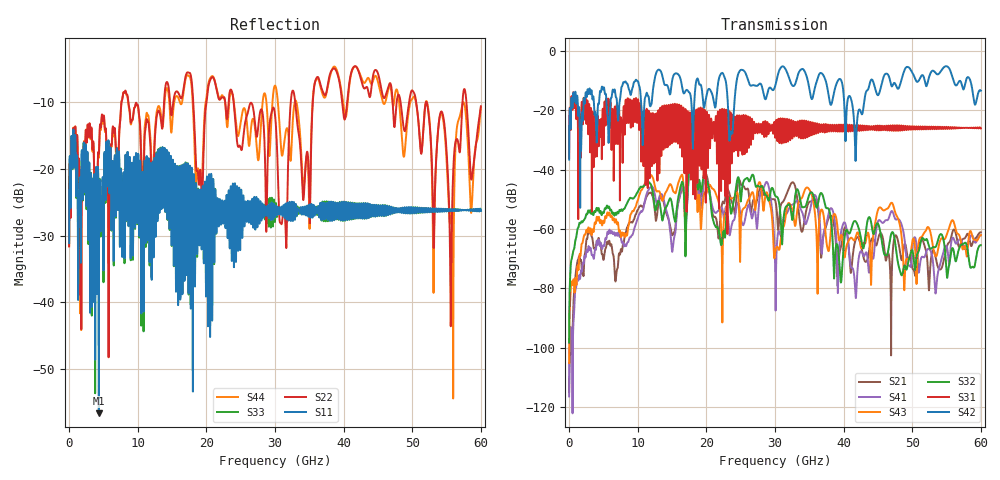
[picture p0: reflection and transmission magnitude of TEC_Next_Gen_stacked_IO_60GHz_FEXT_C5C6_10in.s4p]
!! CHANNEL DESCRIPTION:  Next Generation 28Gbps Press-fit Stacked I/O Connector
!!  with 10" 5-6-5 Megtron 6 Stripline trace on host side and 1.25" 7-5-7 Megtron 6 Microstrip trace on plug side
!! HOST PCB DESCRIPTION:  PCB thickness 3.425 mm
!!  26 Layer Board, 15 GND planes, 4 Layer route-out on Layers 7,11,17,21, 8mil stub on vias
!!  Pairs on following layers
!!  Layer 07 - A02A03 A14A15 D05D06
!!  Layer 11 - D020D3 C05C06 D14D15
!!  Layer 17 - C02C03 B05B06 C14C15
!!  Layer 21 - B02B03 A05A06 B14B15
!! CONNECTOR DESCRIPTION:  Next Generation 28Gbps Press-fit Stacked I/O Connector
!! PLUG-IN CARD DESCRIPTION:  PCB thickness 1mm thick
!!  6 Layer Board, 4 GND planes, 0.35 x 1.4mm mating pads
!!  Micro-strip diff traces referenced to GND plane 3mils down, 2nd GND plane 17mils from top of board
!!  PCB GND planes are symmetric
!! MODEL DESCRIPTION: TE Connectivity S-parameter model produced from Macro-model, Extracted .s4p FEXT (Victim B05B06 - Aggressor C05C06)
!! MODEL DATE: 5/15/2014 CR32f, FPR23
!! MODEL STATUS: Developmental
!! MODEL GEOMETRY: 4 Rows - Rows A, B, C, D. 3 pairs in each row, 12 total pairs
!! MODEL FREQUENCY RANGE: DC to 60 GHz in 10 MHz frequency steps
!! MODEL EDGE RATE LIMITATION: 8.33 ps (Using conservative 0.5/Fmax rule of thumb)
!! TIME-DOMAIN TRANSFORM CAUTIONS:
!! 1.) Do not simulate transient edge rates faster than the number listed above.  Edge
!!  rates faster than this number contain significant spectral content at frequencies
!!  above the model's highest frequency.
!! 2.) Even when simulating edge rates that are slower than the number listed above, be
!!  aware that the best time resolution possible with a direct iFFT is (1 / 2Fmax).
!!  As a result, time resolution is typically not adequate for most time-domain
!!  simulations unless tricks such as frequency-domain zero-padding and windowing are
!!  used to minimize leakage and aliasing.
!! 3.) Because the model has a uniform frequency step, a direct iFFT will result in an
!!  impulse that that has a time length given by either (1 / Fstep) or (1 / 2Fstep),
!!  depending on the transform being used.  Care has been taken in selecting the
!!  frequency step to ensure a settled impulse response for the model.  Therefore,
!!  convolution with the model's impulse response should present no issues.  However,
!!  if directly concatenating s-parameter models in the frequency domain a user must
!!  either interpolate necessary interim frequencies or complete impulse response
!!  zero-padding.  Impulse response zero-padding is more difficult, but more accurate.
!! PORT DEFINITIONS:
!! Port  1  ----->  Host C05		B05 Module <-----  Port  2
!! Port  3  ----->  Host C06		B06 Module <-----  Port  4
!! Touchstone data
! Created: 29-Sep-2014 by IdEM R2011 (7.0.3)
# Hz S MA R 50
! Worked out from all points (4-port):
!   6000 points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, 10 MHz to 60 GHz, reference 50 ohm
!   strongest paths, dB at 10 MHz, 15.01 GHz, 30.01 GHz, 45.01 GHz, 60 GHz:
!     S42: -36.6, -10.1, -12.0, -14.9, -13.4
!     S31: -36.1, -23.7, -27.6, -25.3, -26.1
!     S32: -98.2, -51.7, -48.7, -58.2, -65.4
!     S43: -105.1, -46.0, -68.2, -53.5, -62.0
!     S41: -116.4, -67.6, -70.9, -57.4, -62.1
!     S21: -114.9, -62.0, -50.2, -63.5, -61.1
!   lowest |S11| = -56.6 dB at 4.34 GHz (marker M1), VSWR 1.00, Z = 50 + j0.144 ohm
!   |S11| at or under -10 dB: start of sweep to end of sweep
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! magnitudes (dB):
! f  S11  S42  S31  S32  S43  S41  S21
! 10 MHz  -31.1  -36.6  -36.1  -98.2  -105.1  -116.4  -114.9
! 4.34 GHz  -56.6  -17.8  -30.5  -53.2  -55.9  -63.5  -63.2
! 17.98 GHz  -24.6  -26.6  -22.3  -36.1  -36.1  -37.6  -37.6
! 22.13 GHz  -28.3  -7.7  -32.6  -65.2  -58.3  -52.8  -53.9
! 35.82 GHz  -26.8  -12.3  -24.2  -50.8  -54.5  -48.5  -49.9
! 41.71 GHz  -26.2  -35.7  -26.4  -57.3  -63.0  -81.3  -63.9
! 60 GHz  -26.3  -13.4  -26.1  -65.4  -62.0  -62.1  -61.1
